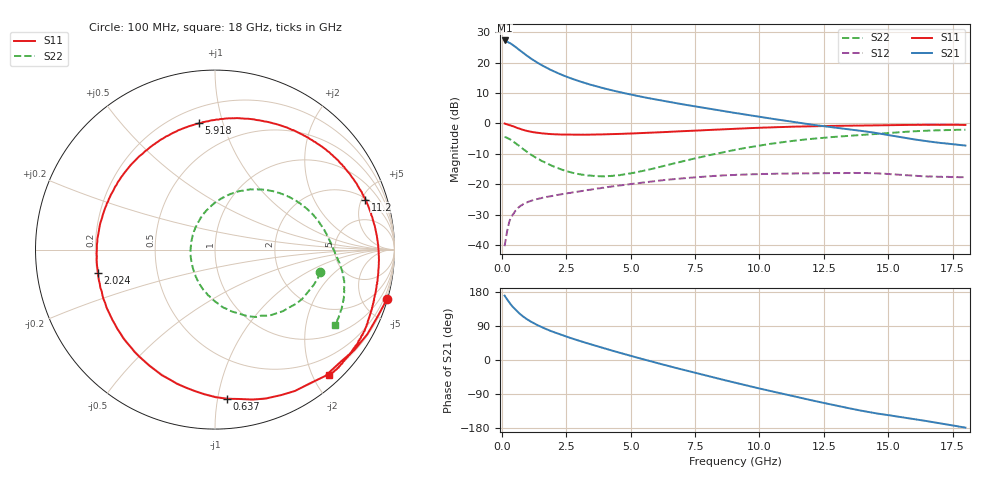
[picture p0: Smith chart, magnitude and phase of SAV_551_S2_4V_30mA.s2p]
! Data provided by Modelithics, Inc.  Tampa, Florida USA, June 2008
!Model SAV-551+
!VAR V_out= 4
!VAR I_out= 30
!VAR V_in= 0.3582
!VAR I_in= 0.8711
!BEGIN ACDATA
# GHZ S MA R 50
! Scattering Parameters
!% F n11x n11y n21x n21y n12x n12y n22x n22y
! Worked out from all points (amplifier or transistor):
!   401 points, 100 MHz to 18 GHz, reference 50 ohm
!   highest |S21| = 27.2 dB at 100 MHz (marker M1)
!   |S21| within 3 dB of that: start of sweep to 655.7 MHz
!   unconditionally stable (mu >= 1): 4.095 GHz to 10.03 GHz; 10.04 GHz to 10.1 GHz; 10.16329 GHz to 10.18275 GHz
!   at 3.054 GHz: K = 0.89, MSG = 18.0 dB, |S12| = -22.2 dB
!   at 9.05 GHz: K = 1.04, MAG = 8.9 dB, |S12| = -16.9 dB
!   at 18 GHz: K = 0.87, MSG = 5.2 dB, |S12| = -17.6 dB
!   lowest NFmin = 0.07 dB at 500 MHz
!   S11 on the Smith chart (normalised r, x): 100 MHz: 0.06, -7.16; 637 MHz: 0.20, -1.06; 2.024 GHz: 0.20, -0.10; 5.918 GHz: 0.30, +0.84; 11.2 GHz: 2.12, +5.35; 18 GHz: 0.17, -2.24
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0.1  0.9979 -15.9  23.03 169.8  0.00969 82.5  0.5983 -12.0
0.1895  0.9709 -29.0  22 160.7  0.01636 74.8  0.5838 -19.8
0.279  0.9392 -41.4  21.09 152.0  0.02424 73.0  0.558 -29.6
0.3685  0.9132 -54.8  20.1 144.1  0.02891 61.5  0.5259 -37.5
0.50275  0.8765 -71.3  18.31 133.9  0.03608 56.5  0.4805 -49.4
0.637  0.8334 -85.5  16.53 125.0  0.04166 48.5  0.4397 -58.7
0.77125  0.7965 -98.0  14.92 117.4  0.04551 43.8  0.3953 -66.8
0.9055  0.7667 -109.1  13.52 110.6  0.04981 40.3  0.3593 -74.3
1.174  0.725 -128.2  11.26 99.2  0.05452 33.8  0.2984 -87.5
1.532  0.6895 -147.7  9.09 87.0  0.05976 29.4  0.2436 -102.3
2.02425  0.6659 -168.6  7.125 73.2  0.06567 23.8  0.1959 -120.2
2.47175  0.6569 176.2  5.927 62.3  0.07064 20.8  0.1671 -135.3
3.09825  0.6537 157.9  4.783 48.6  0.07799 16.2  0.1444 -156.5
4.396  0.6694 127.2  3.398 22.5  0.09457 6.5  0.1396 159.8
5.9175  0.7099 97.2  2.498 -6.0  0.1127 -7.6  0.1835 118.7
6.0965  0.7153 94.0  2.423 -9.1  0.1155 -9.3  0.1925 115.1
7.439  0.7599 71.6  1.925 -32.8  0.1304 -23.0  0.2638 89.2
9.05  0.8157 47.6  1.488 -59.7  0.1428 -40.8  0.3692 63.7
11.198  0.8827 18.4  1.076 -93.9  0.1507 -65.5  0.512 34.2
12.04825  0.8998 8.1  0.9555 -106.6  0.1517 -75.2  0.5602 23.9
15.0465  0.9375 -23.0  0.6416 -146.0  0.1475 -105.8  0.7007 -6.7
18  0.9446 -47.8  0.4336 -178.4  0.1313 -131.1  0.7894 -32.3
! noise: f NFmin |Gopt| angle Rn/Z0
0.5  0.07  0.3651  25.83  0.059
0.7  0.099  0.3711  35.87  0.053
0.9  0.129  0.377  45.79  0.048
1  0.143  0.3799  50.71  0.046
1.9  0.276  0.4052  93.56  0.033
2.4  0.349  0.4185  116.3  0.032
3  0.438  0.4339  142.5  0.036
3.9  0.57  0.4556  179.8  0.053
5  0.732  0.4799  -137.9  0.092
6  0.879  0.5  -102.8  0.145
